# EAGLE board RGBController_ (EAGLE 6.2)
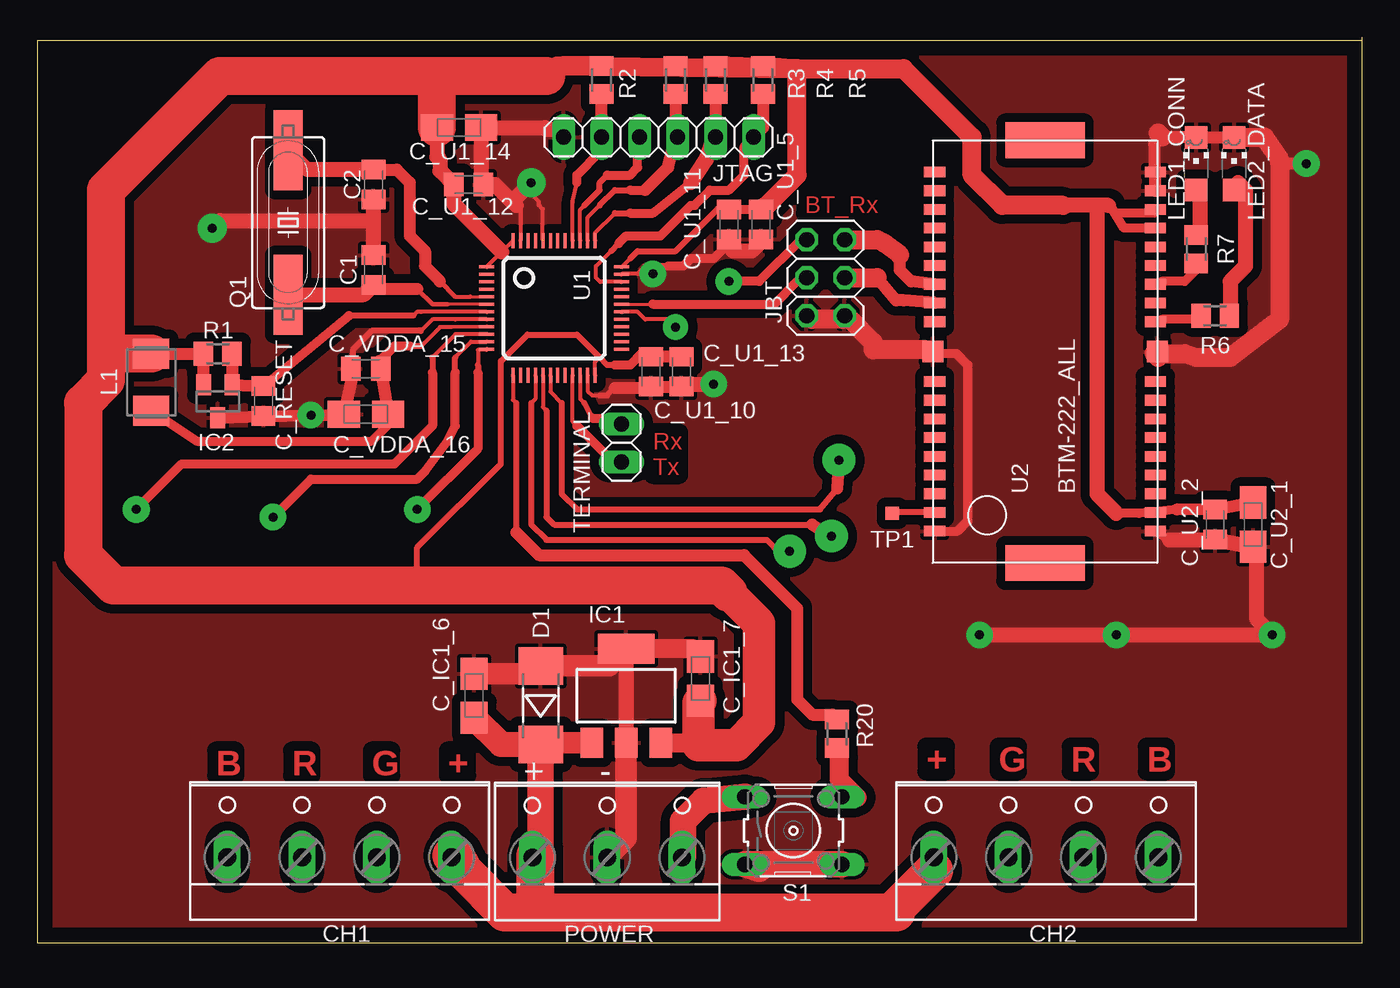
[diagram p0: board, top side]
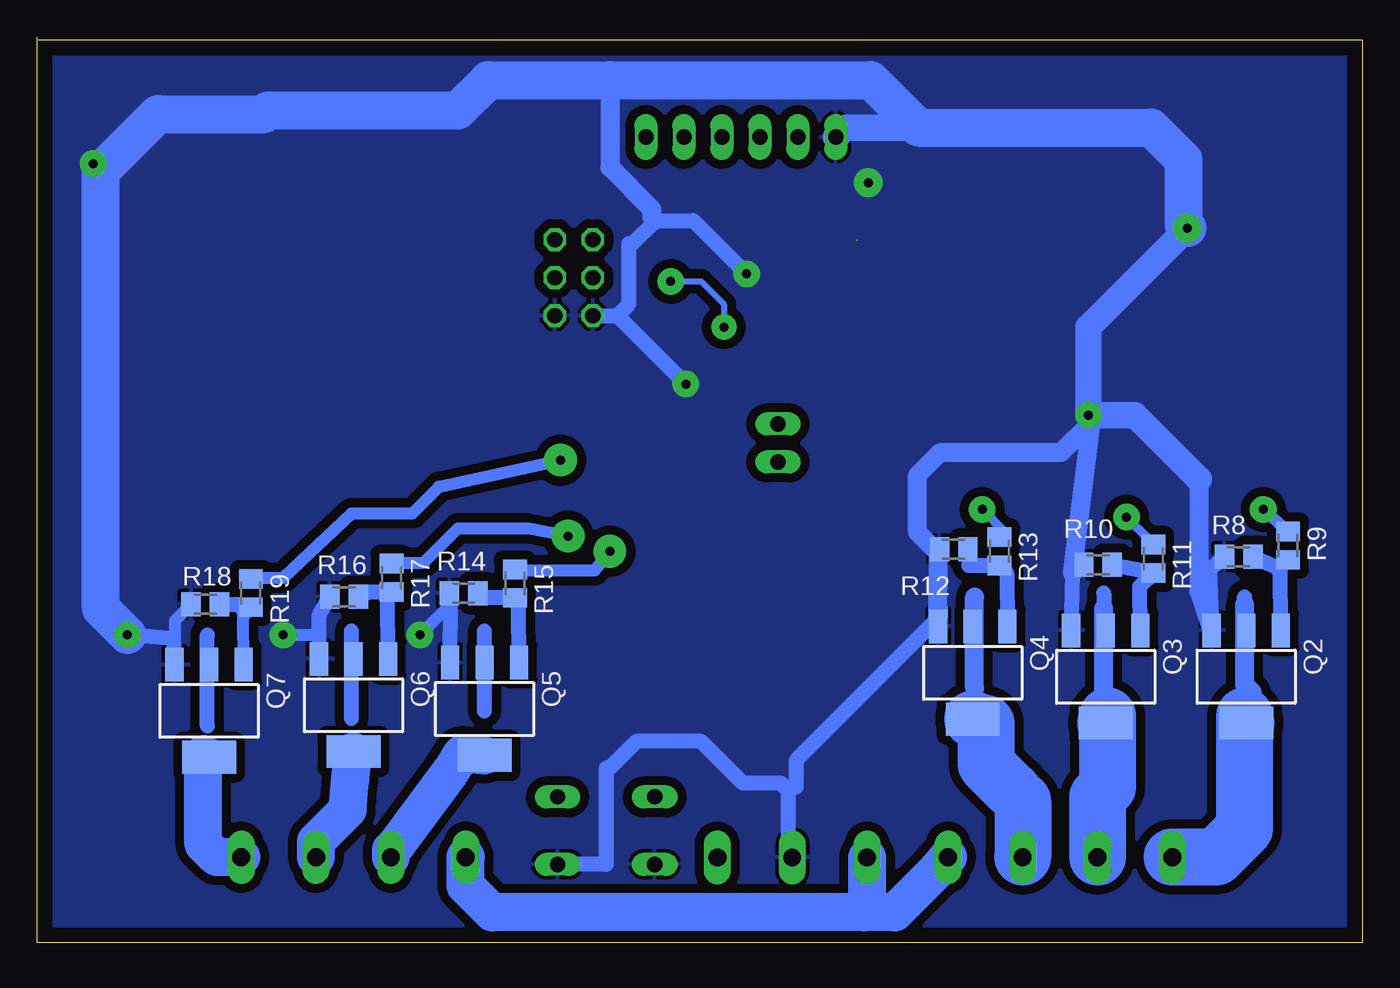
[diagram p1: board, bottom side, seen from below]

Size 88.57 x 60.51 mm. Coordinates in mm from the lower left corner, seen from the top.
Outline: 88.57,60.51 88.57,0 0,0 0,60.33 88.52,60.33
Copper layers (1*16): Top 0.035mm / dielectric 1.5mm / Bottom 0.035mm
Design rules: minimum track width 8mil, minimum drill 15mil, track to track 10mil, track to pad 10mil, pad to pad 10mil, via to via 10mil, smd to smd 8mil, copper to edge 40mil, drill to drill 8mil, minimum pad ring 10mil, minimum via ring 8mil, stop-mask expansion 4mil, vias tented up to drill 0mil, thermal gap 10mil

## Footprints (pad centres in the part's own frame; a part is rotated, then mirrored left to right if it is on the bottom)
C0805K = smd 1.3 x 1.6: 1 -1,0; 2 1,0
A/3216-18W = smd 2.15 x 1.8: + 1.475,0; - -1.475,0
W237-4 = drill 1.194 long: 1 -7.5,-1.27; 2 -2.5,-1.27; 3 2.5,-1.27; 4 7.5,-1.27
MELF-MLL41 = smd 2.5 x 3: A 2.625,0; C -2.625,0
SOT223 = smd 1.5 x 2: 1 -2.3,-3.15; 2 0,-3.15; 3 2.3,-3.15 | smd 3.8 x 2: 4 0,3.15
SOT23 = smd 1 x 1.4: 1 -0.95,-1.1; 2 0.95,-1.1; 3 0,1.1
2X03 = drill 1.016 octagon: 1 -2.54,-1.27; 2 -2.54,1.27; 3 0,-1.27; 4 0,1.27; 5 2.54,-1.27; 6 2.54,1.27
1X06 = drill 1.016 long: 1 -6.35,0; 2 -3.81,0; 3 -1.27,0; 4 1.27,0; 5 3.81,0; 6 6.35,0
L4532M = smd 2 x 2.4: 1 -1.9,0; 2 1.9,0
CHIPLED_1206 = smd 1.5 x 1.5: A 0,-1.75; C 0,1.75
W237-103 = drill 1.194 long: 1 -5,-1.29; 2 0,-1.29; 3 5,-1.29
HC49UP = smd 5.334 x 1.93: 1 -4.826,0; 2 4.826,0
SOT223' = smd 1.219 x 2.235: 1 -2.311,-3.099; 2 0,-3.099; 3 2.311,-3.099 | smd 3.6 x 2.2: 4 0,3.099
M0805 = smd 1.3 x 1.6: 1 -0.95,0; 2 0.95,0
B3F-10XX = drill 1.016 long: 1 -3.251,2.261; 2 3.251,2.261; 3 -3.251,-2.261; 4 3.251,-2.261
1X02 = drill 1.016 long: 1 -1.27,0; 2 1.27,0
TP09SQ = smd 0.9 x 0.9: TP 0,0
TQFP48 = smd 0.2 x 1: 1 -2.75,-4.5; 2 -2.25,-4.5; 3 -1.75,-4.5; 4 -1.25,-4.5; 5 -0.75,-4.5; 6 -0.25,-4.5; 7 0.25,-4.5; 8 0.75,-4.5; 9 1.25,-4.5; 10 1.75,-4.5; 11 2.25,-4.5; 12 2.75,-4.5; 25 2.75,4.5; 26 2.25,4.5; 27 1.75,4.5; 28 1.25,4.5; 29 0.75,4.5; 30 0.25,4.5; 31 -0.25,4.5; 32 -0.75,4.5; 33 -1.25,4.5; 34 -1.75,4.5; 35 -2.25,4.5; 36 -2.75,4.5 | smd 1 x 0.2: 13 4.5,-2.75; 14 4.5,-2.25; 15 4.5,-1.75; 16 4.5,-1.25; 17 4.5,-0.75; 18 4.5,-0.25; 19 4.5,0.25; 20 4.5,0.75; 21 4.5,1.25; 22 4.5,1.75; 23 4.5,2.25; 24 4.5,2.75; 37 -4.5,2.75; 38 -4.5,2.25; 39 -4.5,1.75; 40 -4.5,1.25; 41 -4.5,0.75; 42 -4.5,0.25; 43 -4.5,-0.25; 44 -4.5,-0.75; 45 -4.5,-1.25; 46 -4.5,-1.75; 47 -4.5,-2.25; 48 -4.5,-2.75
BTM-222 = smd 2.4 x 5.3: $AGND -14.625,3.75; $BGND 13.625,3.75 | smd 0.711 x 1.422: P$1 -12.5,-3.625; P$2 -11.25,-3.625; P$3 -10,-3.625; P$4 -8.75,-3.625; P$5 -7.5,-3.625; P$6 -6.25,-3.625; P$7 -5,-3.625; P$8 -3.75,-3.625; P$9 -2.5,-3.625; P$11 1.5,-3.625; P$12 2.75,-3.625; P$13 4,-3.625; P$14 5.25,-3.625; P$15 6.5,-3.625; P$16 7.75,-3.625; P$17 9,-3.625; P$18 10.25,-3.625; P$19 11.5,-3.625; P$20 11.5,11.125; P$21 10.25,11.125; P$22 9,11.125; P$23 7.75,11.125; P$24 6.5,11.125; P$25 5.25,11.125; P$26 4,11.125; P$27 2.75,11.125; P$28 1.5,11.125; P$30 -2.5,11.125; P$31 -3.75,11.125; P$32 -5,11.125; P$33 -6.25,11.125; P$34 -7.5,11.125; P$35 -8.75,11.125; P$36 -10,11.125; P$37 -11.25,11.125; P$38 -12.5,11.125 | smd 1.422 x 1.4: P$10 -0.5,-3.75; P$29 -0.5,11.25

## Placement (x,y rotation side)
C1  22p  [C0805K]  22.48,44.96 270 top
C2  22p  [C0805K]  22.48,50.67 90 top
C_IC1_6  4.7uF  [A/3216-18W]  29.21,16.51 270 top
C_IC1_7  1uF  [A/3216-18W]  44.32,17.65 270 top
C_RESET  100n  [C0805K]  15.11,36.2 90 top
C_U1_5  100n  [C0805K]  48.39,48.01 90 top
C_U1_10  100n  [C0805K]  41.02,38.16 90 top
C_U1_11  100n  [C0805K]  46.23,48.01 90 top
C_U1_12  100n  [C0805K]  28.83,50.67 180 top
C_U1_13  100n  [C0805K]  43.05,38.16 90 top
C_U1_14  4.7uF  [A/3216-18W]  28.19,54.48 180 top
C_U2_1  1uF  [A/3216-18W]  81.28,27.94 90 top
C_U2_2  100n  [C0805K]  78.74,27.94 90 top
C_VDDA_15  10n  [C0805K]  21.97,38.35 0 top
C_VDDA_16  1uF  [A/3216-18W]  21.97,35.31 0 top
CH1  CH1  [W237-4]  20.19,6.99 0 top
CH2  CH2  [W237-4]  67.44,6.99 0 top
D1  1N4007  [MELF-MLL41]  33.66,15.88 90 top
IC1  MCP1825  [SOT223]  39.37,16.51 0 top
IC2  DS1818  [SOT23]  12.06,36.2 180 top
JBT  [2X03]  52.7,44.45 90 top
JTAG  [1X06]  41.53,53.85 180 top
L1  10uH  [L4532M]  7.62,37.47 90 top
LED1_CONN  [CHIPLED_1206]  77.47,52.07 0 top
LED2_DATA  [CHIPLED_1206]  80.01,52.07 0 top
POWER  [W237-103]  38.1,6.99 0 top
Q1  8MHz  [HC49UP]  16.76,48.13 90 top
Q2  IRLR2905PBF  [SOT223']  7.75,17.78 180 bottom
Q3  IRLR2905PBF  [SOT223']  17.14,17.78 180 bottom
Q4  IRLR2905PBF  [SOT223']  26.04,18.03 180 bottom
Q5  IRLR2905PBF  [SOT223']  58.67,15.62 180 bottom
Q6  IRLR2905PBF  [SOT223']  67.44,15.88 180 bottom
Q7  IRLR2905PBF  [SOT223']  77.09,15.49 180 bottom
R1  10k  [M0805]  12.06,39.37 180 top
R2  10k  [M0805]  37.72,57.66 90 top
R3  10k  [M0805]  42.67,57.66 90 top
R4  10k  [M0805]  45.34,57.66 90 top
R5  10k  [M0805]  48.51,57.66 90 top
R6  820  [M0805]  78.74,41.91 0 top
R7  820  [M0805]  77.47,46.35 90 top
R8  10K  [M0805]  8.26,25.78 180 bottom
R9  220  [M0805]  4.95,26.54 270 bottom
R10  10K  [M0805]  17.65,25.27 180 bottom
R11  220  [M0805]  13.97,25.65 270 bottom
R12  10K  [M0805]  27.3,26.29 180 bottom
R13  220  [M0805]  24.26,26.16 270 bottom
R14  10K  [M0805]  60.07,23.37 180 bottom
R15  220  [M0805]  56.64,24 270 bottom
R16  10K  [M0805]  68.07,23.11 180 bottom
R17  220  [M0805]  64.9,24.38 270 bottom
R18  10K  [M0805]  77.34,22.61 180 bottom
R19  220  [M0805]  74.3,23.37 270 bottom
R20  10k  [M0805]  53.47,13.97 270 top
S1  [B3F-10XX]  50.55,7.49 0 top
TERMINAL  [1X02]  39.05,33.4 270 top
TP1  PTR1TP09SQ  [TP09SQ]  57.15,28.7 0 top
U1  STM32F10XCXT6  [TQFP48]  34.54,42.42 270 top
U2  BTM-222_ALL  [BTM-222]  71.12,40.01 90 top

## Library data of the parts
C1 C2 C_RESET C_U1_5 C_U1_10-C_U1_13 C_U2_2 C_VDDA_15 R1-R20 = resistor
C_IC1_6 C_IC1_7 C_U1_14 C_U2_1 C_VDDA_16 L1 = rcl
CH1 CH2 = con-wago-500; OC_FARNELL: unknown; OC_NEWARK: unknown
D1 = diode
IC1 = v-reg
IC2 = maxim; MF: MAXIM; MPN: MAX6520EUR-T; OC_FARNELL: unknown; OC_NEWARK: 02J4586
JBT JTAG TERMINAL = pinhead
LED1_CONN LED2_DATA = led
POWER = con-wago-500; MPN: 237-103; OC_FARNELL: unknown; OC_NEWARK: 18M7116
Q1 = crystal; OC_FARNELL: unknown; OC_NEWARK: unknown
Q2-Q7 = transistor-power
S1 = switch-omron; MPN: B3F-1000; OC_FARNELL: 176432; OC_NEWARK: 36M3542
TP1 = testpad
U1 = stm32
U2 = BTM_222

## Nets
+3V3: C_IC1_7.+ C_U1_5.2 C_U1_10.2 C_U1_11.2 C_U1_12.2 C_U1_13.2 C_U1_14.+ C_U2_1.+ C_U2_2.2 IC1.3 IC2.2 L1.2 R1.2 R2.2 R3.2 R4.2 R5.2 U1.1 U1.24 U1.36 U1.48 U2.P$2 U2.P$16 U2.P$17
BT_RX: JBT.6 U1.30
BT_TX: JBT.4 U1.31
CH1_B: R13.1 U1.12
CH1_G: R11.1 U1.11
CH1_R: R9.1 U1.10
CH2_B: R19.1 U1.18
CH2_G: R17.1 U1.17
CH2_R: R15.1 U1.16
GND: C1.1 C2.1 C_IC1_6.- C_IC1_7.- C_RESET.1 C_U1_5.1 C_U1_10.1 C_U1_11.1 C_U1_12.1 C_U1_13.1 C_U1_14.- C_U2_1.- C_U2_2.1 C_VDDA_15.1 C_VDDA_16.- D1.A IC1.2 IC1.4 IC2.3 JBT.1 JBT.2 JTAG.6 LED1_CONN.C LED2_DATA.C POWER.2 Q2.3 Q3.3 Q4.3 Q5.3 Q6.3 Q7.3 R8.2 R10.2 R12.2 R14.2 R16.2 R18.2 S1.3 S1.4 U1.8 U1.23 U1.35 U1.44 U1.47 U2.P$1 U2.P$10 U2.P$18 U2.P$19 U2.P$29 U2.P$38
N$1: TP1.TP U2.P$37
N$2: LED2_DATA.A R6.2
N$3: R6.1 U2.P$11
N$4: R7.1 U2.P$13
N$5: LED1_CONN.A R7.2
N$6: JBT.3 U2.P$27
N$7: JBT.5 U2.P$26
N$8: TERMINAL.1 U1.22
N$9: TERMINAL.2 U1.21
N$10: Q2.1 R8.1 R9.2
N$12: C_RESET.2 IC2.1 R1.1 U1.7
N$13: CH1.1 Q2.2 Q2.4
N$14: C2.2 Q1.2 U1.5
N$15: JTAG.1 R5.1 U1.34
N$16: JTAG.2 R4.1 U1.37
N$17: JTAG.3 R3.1 U1.38
N$18: JTAG.5 R2.1 U1.40
N$19: JTAG.4 U1.39
N$20: Q3.1 R10.1 R11.2
N$21: Q4.1 R12.1 R13.2
N$24: CH1.2 Q3.2 Q3.4
N$25: CH1.3 Q4.2 Q4.4
N$26: Q5.1 R14.1 R15.2
N$28: Q6.1 R16.1 R17.2
N$29: C1.2 Q1.1 U1.6
N$31: Q7.1 R18.1 R19.2
N$32: CH2.2 Q5.2 Q5.4
N$33: R20.2 S1.2
N$34: CH2.3 Q6.2 Q6.4
N$35: CH2.4 Q7.2 Q7.4
N$37: POWER.3 S1.1
N$47: C_VDDA_15.2 C_VDDA_16.+ L1.1 U1.9
POWER_ON: R20.1 U1.13
V+: C_IC1_6.+ CH1.4 CH2.1 D1.C IC1.1 POWER.1

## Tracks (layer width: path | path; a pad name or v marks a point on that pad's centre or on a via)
+3V3
  Top 0.254: U1.48 31.05,46.17 U1.1 | U1.36 39.07,45.17 39.62,45.72 | U1.24 37.29,38.82 37.59,39.12
  Top 0.406: 39.62,45.72 40.13,46.23 42.67,46.23 45.47,49.02 46.75,49.02 C_U1_11.2 | 46.23,23.37 29.97,23.37 29.46,23.88 26.42,23.88 25.4,24.89 25.4,26.42 30.99,32 30.99,38.86 32.77,40.64 36.07,40.64 37.59,39.12 38.1,38.61 38.61,38.61
  Top 0.61: C_U1_11.2 C_U1_5.2 | C_U1_10.2 40.43,39.42 39.62,38.61 38.61,38.61 | 71.88,49.02 72.14,48.77 74.68,48.77 U2.P$17 | 71.88,49.02 71.63,49.28 | U2.P$2 76.2,28.96 73.66,28.7 72.14,28.7 | U2.P$16 73.41,47.75 72.64,47.75 71.88,49.02
  Top 0.813: IC2.2 R1.2 L1.2 | C_U1_13.2 C_U1_10.2 | C_U2_1.+ C_U2_2.2 76.2,28.96
  Top 1.016: C_U1_14.+ 26.72,52.53 26.92,52.32 26.92,51.58 C_U1_12.2 27.83,49.39 31.05,46.17 | R3.2 R2.2 | 34.73,58.61 34.04,57.91 | 71.63,49.28 70.87,49.28 | 70.87,49.28 68.58,49.28 | 72.14,28.7 70.87,29.97 70.87,49.28
  Top 1.27: IC1.3 44.04,13.36 44.2,13.21 | 68.58,49.28 64.52,49.28 62.48,51.31 62.48,53.85 57.91,58.42 50.8,58.42 | C_U1_5.2 48.77,49.28 50.8,51.31 50.8,58.42 | 34.73,58.61 35.05,58.6 | 35.05,58.6 50.8,58.42 | 50.8,58.42 R4.2 | R5.2 50.8,58.42 | R2.2 35.05,58.6
  Top 2.184: 46.23,23.37 48.26,21.34 48.26,14.73 46.74,13.21 44.2,13.21 44.2,16.05 C_IC1_7.+
  Top 2.54: 34.04,57.91 26.42,57.91 | 26.42,57.91 12.19,57.91 4.57,50.29 4.57,39.62 | 4.57,39.62 4.57,37.59 3.05,36.07 3.05,25.91 5.08,23.88 29.46,23.88 45.72,23.88 46.23,23.37 | L1.2 4.83,39.37 4.57,39.62 | C_U1_14.+ 26.72,57.61 26.42,57.91
BT_RX  (via drill 0.6 pad 1.68, 0.6 pad 1.78)
  Top 0.254: v42.67,41.15 42.16,41.66 40.64,41.66 40.13,42.16 39.12,42.16 U1.30
  Top 0.61: JBT.6 51.05,46.99 48.26,44.2 v46.23,44.2
  Bottom 0.406: v42.67,41.15 42.67,42.67 44.2,44.2 v46.23,44.2
BT_TX
  Top 0.203: U1.31 41.15,42.67
  Top 0.61: 41.15,42.67 49.28,42.67 50.8,44.2 51.18,44.2 JBT.4
CH1_B  (via drill 0.6 pad 1.78)
  Top 0.254: U1.12 30,39.62 29.46,39.62 29.46,38.61
  Top 0.406: 29.46,38.61 29.46,38.1
  Top 0.61: 29.46,38.1 29.46,33.02 v25.4,28.96
  Bottom 0.61: v25.4,28.96 23.88,27.43 R13.1
CH1_G  (via drill 0.6 pad 1.78)
  Top 0.254: 27.94,39.12 28.99,40.17 U1.11
  Top 0.406: 27.94,38.1 27.94,39.12
  Top 0.61: v15.75,28.45 18.29,30.99 25.4,30.99 25.91,31.5 27.43,33.53 27.94,34.54 27.94,38.1
  Bottom 0.61: v15.75,28.45 14.22,26.92 R11.1
CH1_R  (via drill 0.6 pad 1.78)
  Top 0.254: U1.10 27.94,40.67 27.94,40.64 26.42,39.12
  Top 0.406: 26.42,39.12 26.42,38.1
  Top 0.61: v6.6,28.96 9.65,32 23.88,32 26.42,34.54 26.42,38.1
  Bottom 0.813: R9.1 v6.6,28.96
CH2_B  (via drill 0.6 pad 2.18)
  Top 0.254: U1.18 34.29,36.83 35.05,36.07
  Top 0.406: 35.05,36.07 35.05,29.97 36.07,28.96 52.32,28.96 53.47,30.35 53.59,31.5
  Top 0.813: v53.59,32.26 53.47,30.35
  Bottom 0.813: v53.59,32.26 61.72,30.48 63.5,28.7 67.56,28.7 72.14,24.38 74.17,24.38 R19.1
CH2_G  (via drill 0.6 pad 2.18)
  Top 0.254: U1.17 33.79,35.8 34.04,35.56
  Top 0.406: 34.04,35.56 34.04,28.45 34.54,27.94 51.82,27.94
  Top 0.813: 51.82,27.94 v53.09,27.18
  Bottom 0.813: R17.1 64.77,25.4 62.74,25.4 60.45,27.69 55.88,27.69 v53.09,27.18
CH2_R  (via drill 0.6 pad 2.18)
  Top 0.254: U1.16 33.29,36.34 33.02,36.07
  Top 0.406: 33.02,36.07 33.02,27.94 34.04,26.92 48.77,26.92 49.66,26.04
  Top 0.813: 49.66,26.04 v50.29,26.16
  Bottom 0.813: v50.29,26.16 51.31,24.89 56.9,24.89 R15.1
GND  (via drill 0.6 pad 1.78, 0.6 pad 1.93)  (1 unrouted)
  Top 0.254: 32,49.28 32.29,48.99 U1.47 | U1.8 27.94,41.66 26.42,41.66 25.65,40.89 | 40.64,45.21 40.13,44.7 39.08,44.7 U1.35 | U1.23 36.79,36.87 37.08,36.58 37.59,36.58 | 33.78,46.99 33.78,49.02 33.53,49.28 33.53,49.53 32.77,50.29 v33.02,50.8
  Top 0.406: 25.65,40.89 22.35,40.89 21.08,39.62 21.08,38.1 21.08,37.85 | 42.16,45.21 41.15,45.21 | 41.15,45.21 40.64,45.21 | 37.59,36.58 38.1,36.58 38.61,37.08 | v41.15,44.7 41.15,45.21
  Top 0.61: C_U1_11.1 45.99,46.5 45.21,45.72 43.69,45.72 43.18,45.21 42.16,45.21 | U2.P$1 75.69,26.92 | U2.P$38 61.54,27.5 62.23,28.19 62.23,38.61 61.47,39.37 60.01,39.37 U2.P$29
  Top 0.813: C_VDDA_15.1 21.08,38.1 | IC2.3 C_RESET.1 v18.29,35.26 C_VDDA_16.- 21.08,37.85 | 38.61,37.08 40.69,37.08 C_U1_10.1 C_U1_13.1 | LED2_DATA.C 79.76,53.85 77.72,53.85 LED1_CONN.C 77.22,53.85 75.18,53.85 74.68,53.34 74.68,51.82 U2.P$19 U2.P$18 | v84.84,52.07 83.06,52.07
  Top 1.016: C1.1 22.48,48.26 | 22.48,48.26 C2.1 | 31.75,49.53 30.61,50.67 C_U1_12.1 29.67,50.83 C_U1_14.- 33.91,54.48 34.04,54.36 34.67,54.36 JTAG.6 | 31.75,49.53 32,49.28 | C_U1_5.1 48.39,46.86 47.75,46.23 46.5,46.23 C_U1_11.1 | 18.29,35.56 v18.29,35.26 | 22.48,48.26 12.19,48.26 v11.68,47.75 | v33.02,50.8 31.75,49.53 | 75.69,26.92 C_U2_2.1 C_U2_1.- 81.53,26.21 81.53,21.59 v82.55,20.57 v72.14,20.57 v62.99,20.57 | IC1.4 IC1.2 | v45.21,37.34 43.43,37.34 C_U1_13.1
  Top 1.27: U2.P$29 59.44,39.62 55.88,39.62 55.88,40.13 54.36,41.66 JBT.1 53.85,41.66 51.82,41.66 JBT.2 | C_IC1_7.- 43.79,19.66 IC1.4 | 74.93,54.1 75.18,53.85 | LED2_DATA.C 80.26,53.85 82.04,53.85 83.06,52.32 83.06,52.07 83.06,41.66 79.76,39.12 77.47,39.12 76.71,39.37 75.18,39.37 74.93,39.12 74.68,39.37 U2.P$10
  Top 1.422: IC1.4 38.21,18.5 D1.A 33.14,17.98 C_IC1_6.- | POWER.2 39.37,6.96 IC1.2
  Top 1.778: S1.4 S1.3 48.26,4.93
  Bottom 0.813: Q7.3 79.37,21.53 R18.2 | R14.2 60.77,22.8 v62.99,20.57 | v72.14,20.57 69.82,20.57 Q6.3 | v84.84,52.07 84.33,51.56 | 72.39,55.63 73.41,55.37
  Bottom 1.016: Q6.3 69.72,21.91 R16.2 | Q5.3 60.95,22.93 R14.2 | R8.2 10.22,24.93 Q2.3 | R10.2 19.36,24.67 Q3.3 | R12.2 28.32,25.21 Q4.3 28.19,22.35 28.19,21.84 37.85,12.19 37.85,10.41 38.1,10.41 38.35,10.16 | POWER.2 38.35,5.95 38.35,10.16 | 38.35,10.16 38.86,10.67 41.4,10.67 44.2,13.46 48.51,13.46 50.29,11.68 50.55,11.68 50.55,5.23 S1.4 | JBT.2 49.78,41.91 | 49.78,41.91 49.02,42.67 49.02,46.74 48.77,46.74 47.24,48.26 44.7,48.26 v41.15,44.7 | 49.78,41.91 v45.21,37.34 | Q7.3 79.5,20.32 v82.55,20.57
  Bottom 1.27: 10.92,30.99 10.92,23.48 Q2.3 | 19.36,24.67 18.09,34.8 | 18.09,34.8 18.09,35.06 v18.29,35.26 | Q4.3 28.32,26.03 29.72,27.43 29.72,31.24 28.19,32.77 20.13,32.77 18.09,34.8 | 50.29,57.66 50.29,51.82 47.5,49.02 47.5,48.51 47.24,48.26
  Bottom 1.778: C_U1_14.- 34.54,54.48 JTAG.6 | v11.68,47.75 18.29,41.14 v18.29,35.26 15.2,35.26 10.92,30.99
  Bottom 2.54: v82.55,20.57 84.33,22.35 84.33,51.56 80.52,55.37 73.41,55.37 | 73.15,55.63 72.39,55.63 60.45,55.63 58.42,57.66 50.29,57.66 32.84,57.66 C_U1_14.- 14.1,54.48 11.94,52.32 11.94,48.01 v11.68,47.75
  pour Bottom (isolate 0.61): -0.51,60.71 88.9,60.71 88.9,-0.51 -0.51,-0.51
  pour Top (isolate 0.61): 0,60.71 -0.25,60.71 -0.25,-0.25 89.15,-0.25 89.15,60.45 0,60.45
N$1
  Top 0.406: U2.P$37 57.15,28.75 TP1.TP
N$2
  Top 1.016: R6.2 79.76,42.16 79.76,44.2 80.77,45.21 80.77,50.29 80.26,50.8 LED2_DATA.A
N$3
  Top 0.61: U2.P$11 75.18,41.66 77.72,41.66 R6.1
N$4
  Top 0.61: R7.1 77.72,45.21 76.71,44.2 75.18,44.2 U2.P$13
N$5
  Top 1.016: R7.2 77.72,47.75 77.72,50.29 LED1_CONN.A
N$6
  Top 0.813: U2.P$27 57.91,42.93 57.4,42.93 56.13,44.45
  Top 1.27: JBT.3 56.13,44.45
N$7
  Top 0.813: U2.P$26 58.42,44.2 57.66,44.96 57.66,45.97
  Top 1.27: 57.66,45.97 56.64,46.74 56.13,46.99 JBT.5
N$8
  Top 0.254: U1.22 36.29,36.35 36.58,36.07
  Top 0.406: 36.58,36.07 37.08,35.05
  Top 0.61: 37.08,35.05 38.42,35.05 TERMINAL.1
N$9
  Top 0.254: U1.21 35.79,34.82 36.07,34.54
  Top 0.61: TERMINAL.2 37.97,32.64 36.07,34.54
N$10
  Bottom 1.016: Q2.1 5.47,25.08 | 5.47,25.08 R9.2 | R8.1 5.53,25.02 5.47,25.08
N$12
  Top 0.254: U1.7 25.66,42.17 25.65,42.16 25.4,42.16 25.15,41.91
  Top 0.406: 25.15,41.91 20.83,41.91
  Top 0.61: 20.83,41.91 C_RESET.2
  Top 0.813: R1.1 IC2.1 C_RESET.2
N$13
  Bottom 3.81: Q2.4 7.87,15.15 7.87,7.62 9.78,5.71 CH1.1
N$14
  Top 0.203: 28.96,43.18 U1.5
  Top 0.254: 27.94,43.18 28.96,43.18
  Top 0.305: 26.92,44.2 27.94,43.18
  Top 0.813: C2.2 24.02,51.67 24.89,50.8 24.89,47.24 25.91,46.23 25.91,45.21 26.92,44.2
  Top 1.016: C2.2 18.05,51.67 Q1.2
N$15
  Top 0.254: U1.34 37.62,44.17 37.34,44.45 37.34,45.21 38.35,46.23
  Top 0.406: 38.35,46.23 38.86,46.74
  Top 0.61: 38.86,46.74 39.37,47.24 41.66,47.24 43.69,49.28 43.94,49.28 44.96,50.29 46.23,50.29 47.24,51.31 47.24,53.21 JTAG.1
  Top 0.813: R5.1 48.51,54.48 JTAG.1
N$16
  Top 0.254: U1.37 37.29,47.45 38.61,48.77
  Top 0.406: 38.61,48.77 39.62,48.77
  Top 0.61: 39.62,48.77 41.15,48.77 43.69,50.8
  Top 0.813: R4.1 JTAG.2
  Top 1.016: 43.69,50.8 44.7,52.32 45.21,53.72 JTAG.2
N$17
  Top 0.254: U1.38 36.79,48.48 37.59,49.28
  Top 0.406: 37.59,49.28 38.61,50.29 39.62,50.29
  Top 0.61: 39.62,50.29 40.64,50.29
  Top 0.813: R3.1 42.35,56.71 42.67,56.39 42.67,53.98 JTAG.3 42.67,53.72 42.16,51.82 40.64,50.29
N$18
  Top 0.254: U1.40 35.79,49.51 36.07,50.8
  Top 0.61: 36.07,50.8 36.07,51.31 37.59,52.83 37.59,53.72 JTAG.5
  Top 0.813: JTAG.5 R2.1
N$19
  Top 0.254: U1.39 36.29,48.99 36.58,49.28
  Top 0.406: 36.58,49.28 37.59,50.29 37.59,50.8 38.1,51.31
  Top 0.61: 38.1,51.31 39.62,51.31 40.13,51.82 40.13,53.72 JTAG.4
N$20
  Bottom 1.016: Q3.1 14.87,23.81 R11.2 14.03,24.77 R10.1
N$21
  Bottom 1.016: Q4.1 23.75,24.71 R13.2 26.29,25.21 R12.1
N$24
  Bottom 2.184: 17.02,10.41 17.69,9.74
  Bottom 3.81: Q3.4 17.02,15.15 17.02,10.41 | 17.69,9.74 CH1.2
N$25
  Bottom 2.184: 23.37,10.16 22.69,9.48
  Bottom 3.81: Q4.4 25.15,14.64 25.15,11.94 23.37,10.16 | 22.69,9.48 CH1.3
N$26
  Bottom 1.016: Q5.1 56.39,22.55 R15.2 58.81,23.05 R14.1
N$27
  Bottom 1.27: 7.37,16.76 7.87,17.27 7.87,20.07 7.87,20.57 7.87,22.61
N$28
  Bottom 1.016: Q6.1 65.16,23.17 R17.2 66.29,23.43 R16.1
N$29
  Top 0.203: U1.6 27.44,42.67 27.43,42.67
  Top 0.305: 27.43,42.67 26.42,42.67 25.4,43.69
  Top 0.813: 25.4,43.69 22.75,43.69 C1.2
  Top 1.016: Q1.1 21.83,43.31 C1.2
N$30
  Bottom 1.016: 17.27,23.37 17.27,22.1
  Bottom 1.27: 17.27,16.26 17.27,22.1 17.27,22.35
N$31
  Bottom 0.813: Q7.1 74.81,21.9 74.64,22.07 R19.2
  Bottom 1.016: R18.1 75.18,22.61 74.64,22.07
N$32
  Bottom 2.54: CH2.2 64.94,6.18 64.52,6.6 60.96,11.43 60.2,12.61 Q5.4
N$33
  Top 1.27: R20.2 53.59,12.89 53.59,10.92 54.81,9.7 S1.2
N$34
  Bottom 2.54: CH2.3 69.94,6.77 67.82,8.89 67.65,10.88 Q6.4
N$35
  Bottom 2.54: CH2.4 76.58,5.71 77.47,6.6 77.47,12.61 Q7.4
N$36
  Bottom 1.27: 25.91,17.02 25.91,23.11
N$37
  Top 1.778: POWER.3 43.18,5.78 43.18,8.13 44.55,9.5 S1.1
N$38
  Bottom 1.016: 7.87,22.86 7.87,23.11
N$39
  Bottom 1.016: 58.67,15.49 58.67,20.83
N$40
  Bottom 1.016: 67.56,14.99 67.56,20.83
N$41
  Bottom 1.016: 77.22,14.48 77.22,20.57
N$47
  Top 0.254: U1.9 27.69,41.15 26.92,41.15 25.65,39.88
  Top 0.406: 25.65,39.88 24.89,39.88
  Top 0.61: 24.89,39.88 23.88,39.88 22.86,38.86 | L1.1 10.67,33.53 22.35,33.53 23.37,34.54 C_VDDA_16.+ | C_VDDA_15.2 22.92,38.62
  Top 0.813: 22.86,38.86 22.92,38.62 C_VDDA_16.+
POWER_ON
  Top 0.254: U1.13 31.79,36.28 32,36.07
  Top 0.406: 32,36.07 32,27.43 | 53.15,15.24 R20.1
  Top 0.813: 32,27.43 33.53,25.91 47.24,25.91 50.8,22.35 50.8,16.26 51.82,15.24 53.15,15.24
V+
  Top 0.254: POWER.1 33.02,5.84 33.27,5.84 | 27.94,5.84 CH1.4
  Top 1.422: D1.C 33.77,13.36 IC1.1
  Top 1.676: C_IC1_6.+ 31,13.25 D1.C
  Top 1.778: POWER.1 33.66,6.25 D1.C
  Top 2.54: 27.69,5.84 27.94,5.84 28.45,4.83 31.24,2.03 57.4,2.03 57.4,2.29 59.94,4.83 | 33.27,5.84 33.27,2.29
  Bottom 2.54: CH1.4 28.57,4.7 31.24,2.03 33.27,2.03 | 33.27,2.03 58.17,2.03 59.94,3.81 CH2.1 | POWER.1 33.1,2.21 33.27,2.03

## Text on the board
Top: BT_Rx | Rx / Tx | B | R | G | + | + | G | R | B
tNames: + | -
